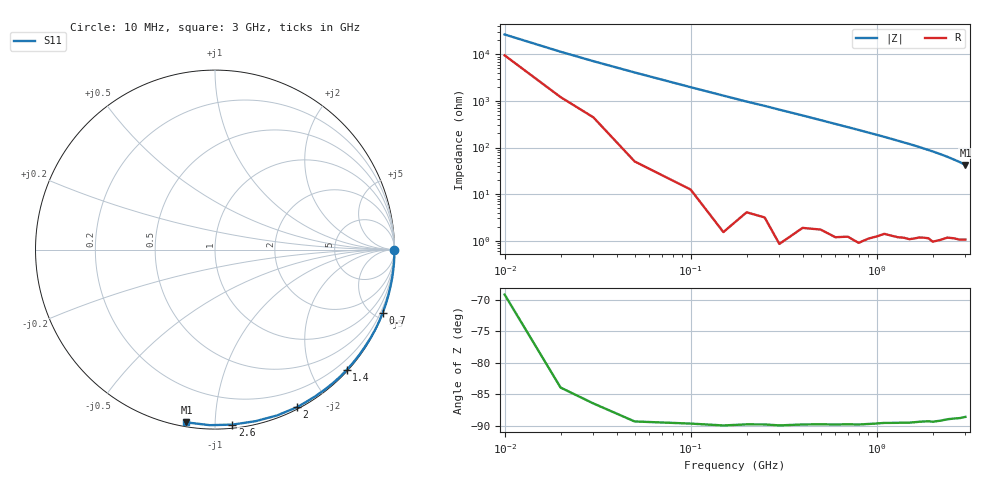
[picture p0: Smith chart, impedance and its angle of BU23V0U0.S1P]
! SIEMENS Small Signal Semiconductors
! BB833
! Si Tuning Diode in SOD323
! VR = 23 V
! S-Parameters:  April  1996
# GHz  S  MA  R  50
!  f  S11
! GHz  MAG  ANG
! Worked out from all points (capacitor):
!   31 points, 10 MHz to 3 GHz, reference 50 ohm
!   read as one part to ground: C = 702 fF near 10 MHz
!   lowest |Z| = 42.4 ohm at 3 GHz (marker M1)
!   S11 on the Smith chart (normalised r, x): 10 MHz: open; 700 MHz: 0.02, -5.48; 1.4 GHz: 0.02, -2.57; 2 GHz: 0.02, -1.65; 2.6 GHz: 0.02, -1.10; 3 GHz: 0.02, -0.85
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0.01  0.9987 -0.2
0.05  0.9997 -1.4
0.15  0.9999 -4.4
0.2  0.9996 -5.9
0.25  0.9995 -7.3
0.3  0.9998 -8.8
0.4  0.9992 -11.7
0.5  0.9989 -14.7
0.6  0.9989 -17.7
0.7  0.9984 -20.7
0.8  0.9985 -23.7
0.9  0.9976 -26.8
1  0.9968 -29.8
1.1  0.9955 -32.9
1.2  0.9951 -36.1
1.3  0.9947 -39.3
1.4  0.994 -42.5
1.5  0.9936 -45.6
1.6  0.9924 -48.9
1.7  0.991 -52.2
1.8  0.99 -55.7
1.9  0.9891 -59.1
2  0.9898 -62.5
2.2  0.9866 -69.5
2.4  0.9823 -76.7
2.6  0.98 -84.3
2.8  0.9786 -91.7
3  0.9757 -99.4
